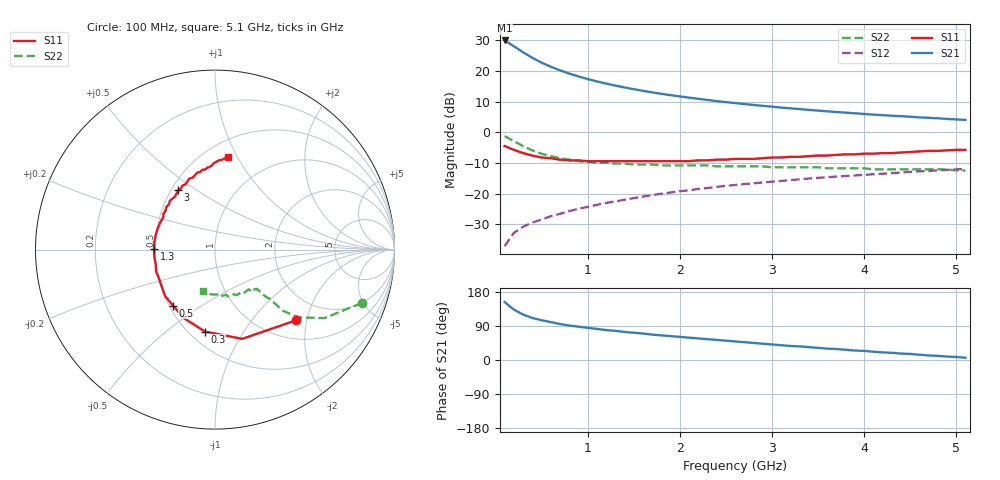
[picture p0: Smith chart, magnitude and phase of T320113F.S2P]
!AT-32011
!S PARAMETERS at Vce=2.7 V  Ic=15mA.  LAST UPDATED 01-05-95
# ghz s ma r 50
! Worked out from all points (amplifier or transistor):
!   51 points, 100 MHz to 5.1 GHz, reference 50 ohm
!   highest |S21| = 30.0 dB at 100 MHz (marker M1)
!   |S21| within 3 dB of that: start of sweep to 256.8 MHz
!   unconditionally stable (mu >= 1): 1.093 GHz to 4.674 GHz
!   at 900 MHz: K = 0.95, MSG = 21.6 dB, |S12| = -24.9 dB
!   at 2.6 GHz: K = 1.07, MAG = 11.7 dB, |S12| = -17.1 dB
!   at 5.1 GHz: K = 0.99, MSG = 8.0 dB, |S12| = -11.9 dB
!   S11 on the Smith chart (normalised r, x): 100 MHz: 1.41, -1.73; 300 MHz: 0.60, -0.69; 500 MHz: 0.52, -0.38; 1.3 GHz: 0.49, +0.01; 3 GHz: 0.54, +0.42; 5.1 GHz: 0.65, +0.91
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0.1  0.6 -41.0  31.53 153.0  0.014 73.0  0.87 -20.0
0.2  0.52 -73.0  25.39 133.0  0.023 64.0  0.72 -32.0
0.3  0.46 -97.0  20.24 120.0  0.029 60.0  0.6 -39.0
0.4  0.42 -114.0  16.49 111.0  0.034 58.0  0.51 -42.0
0.5  0.39 -127.0  13.74 105.0  0.038 58.0  0.45 -42.0
0.6  0.38 -137.0  11.78 100.0  0.043 59.0  0.41 -42.0
0.7  0.36 -146.0  10.28 95.0  0.047 59.0  0.38 -43.0
0.8  0.35 -154.0  9.12 91.0  0.052 60.0  0.36 -43.0
0.9  0.35 -160.0  8.18 88.0  0.057 60.0  0.34 -43.0
1  0.34 -166.0  7.42 85.0  0.061 61.0  0.33 -43.0
1.1  0.34 -171.0  6.79 82.0  0.066 61.0  0.32 -43.0
1.2  0.34 -176.0  6.26 79.0  0.071 61.0  0.32 -44.0
1.3  0.34 179.0  5.8 77.0  0.075 61.0  0.31 -45.0
1.4  0.34 175.0  5.41 74.0  0.08 61.0  0.31 -46.0
1.5  0.34 171.0  5.07 72.0  0.085 61.0  0.3 -46.0
1.8  0.34 159.0  4.26 65.0  0.1 59.0  0.29 -50.0
2.2  0.35 145.0  3.53 57.0  0.12 57.0  0.29 -55.0
2.6  0.37 133.0  3.01 49.0  0.139 54.0  0.28 -61.0
3  0.39 122.0  2.63 41.0  0.158 51.0  0.27 -67.0
3.5  0.42 110.0  2.27 32.0  0.182 46.0  0.27 -75.0
4.3  0.46 94.0  1.87 19.0  0.217 40.0  0.25 -88.0
5.1  0.52 82.0  1.6 6.0  0.254 31.0  0.24 -106.0
